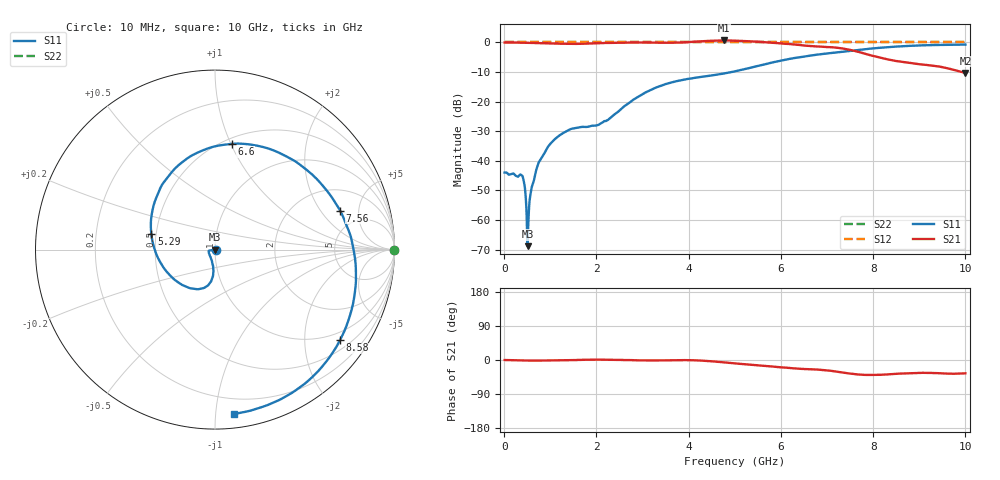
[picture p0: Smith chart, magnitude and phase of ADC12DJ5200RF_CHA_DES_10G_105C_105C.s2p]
! Texas Instruments, Inc.
! ADC12DJ5200RF - CH A S-Parameters (DES Mode, Fs = 10 GSPS, 105 degC case, 105 degC juntion)
! Port 1 represents the 100-ohm differenal input, Port 2 the digital output
! freq  dbS11  angS11  dbS21 angS21 dbS12 angS12 dbS22 angS22
# HZ S DB R 100
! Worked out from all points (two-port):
!   1000 points, 10 MHz to 10 GHz, reference 100 ohm
!   highest |S21| = 0.69 dB at 4.77 GHz (marker M1); lowest = -10.3 dB at 10 GHz (marker M2)
!   |S21| within 3 dB of the highest: start of sweep to 7.437 GHz
!   lowest |S11| = -68.9 dB at 510 MHz (marker M3), VSWR 1.00, Z = 100 - j0.0713 ohm
!   |S11| at or under -10 dB: start of sweep to 4.932 GHz
!   |S22| runs from 0.0 to 0.0 dB; largest |S21 - S12| = 0.77
!   S11 on the Smith chart (normalised r, x): 10 MHz: 1.01, -0.00; 5.29 GHz: 0.47, +0.10; 6.6 GHz: 0.55, +1.01; 7.56 GHz: 3.35, +3.13; 8.58 GHz: 0.75, -2.91; 10 GHz: 0.09, -1.12
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1e7  -43.98 -7.6  0.00 -0.0  0.00 0.0  0.00 0.0
3.8e8  -44.92 -10.5  -0.06 -1.2  0.00 0.0  0.00 0.0
4.3e8  -47.24 -0.5  -0.08 -1.4  0.00 0.0  0.00 0.0
4.7e8  -52.81 6.8  -0.10 -1.4  0.00 0.0  0.00 0.0
5.1e8  -68.87 -81.6  -0.11 -1.5  0.00 0.0  0.00 0.0
6e8  -48.82 -136.8  -0.15 -1.6  0.00 0.0  0.00 0.0
7.1e8  -42.37 -157.4  -0.22 -1.6  0.00 0.0  0.00 0.0
9.4e8  -35.52 -169.1  -0.30 -1.5  0.00 0.0  0.00 0.0
1.26e9  -30.80 -171.7  -0.43 -1.0  0.00 0.0  0.00 0.0
1.68e9  -28.56 -163.4  -0.44 0.4  0.00 0.0  0.00 0.0
2.24e9  -26.25 -119.8  -0.15 0.6  0.00 0.0  0.00 0.0
3.34e9  -14.98 -96.9  -0.09 -1.2  0.00 0.0  0.00 0.0
4.77e9  -10.47 -157.8  0.69 -6.3  0.00 0.0  0.00 0.0
5.01e9  -9.74 -174.4  0.62 -9.0  0.00 0.0  0.00 0.0
5.29e9  -8.74 165.9  0.41 -11.8  0.00 0.0  0.00 0.0
5.9e9  -6.49 126.2  -0.17 -18.2  0.00 0.0  0.00 0.0
6.6e9  -4.49 81.1  -1.13 -24.1  0.00 0.0  0.00 0.0
6.67e9  -4.33 76.5  -1.22 -24.6  0.00 0.0  0.00 0.0
7.56e9  -2.73 17.4  -2.71 -36.8  0.00 0.0  0.00 0.0
8.34e9  -1.56 -25.8  -5.80 -37.8  0.00 0.0  0.00 0.0
8.58e9  -1.31 -35.9  -6.43 -35.9  0.00 0.0  0.00 0.0
1e10  -0.71 -83.2  -10.29 -35.2  0.00 0.0  0.00 0.0
